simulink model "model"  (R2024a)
settings: Solver=VariableStepAuto  StartTime=0.0  StopTime=7*3600  RelTol=1e-3
libraries: fl_lib x8, nesl_utility x2, batteryecm_lib x1

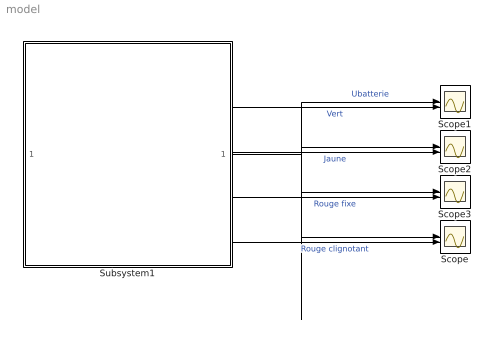
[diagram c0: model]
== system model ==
  Scope{,1..3} (4 alike) : Scope  NumInputPorts=2
  Subsystem1 : Subsystem  mask{U=0, Q=0}
      mask prompts: U "Tension batterie (V)"; Q "Capacité A.h)"
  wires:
  Subsystem1/1(Ubatterie) -> Scope1/1, Scope/1, Scope3/1, Scope2/1  "Ubatterie"
  Subsystem1/2(Vert) -> Scope1/2  "Vert"
  Subsystem1/3(Jaune) -> Scope2/2  "Jaune"
  Subsystem1/4(Rouge fixe) -> Scope3/2  "Rouge fixe"
  Subsystem1/5(Rouge clignotant) -> Scope/2  "Rouge clignotant"

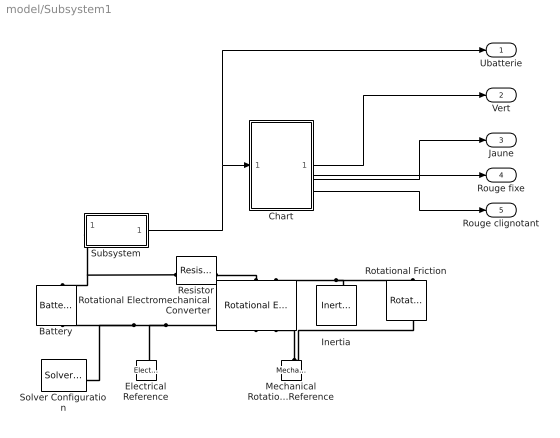
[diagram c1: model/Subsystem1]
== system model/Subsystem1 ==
  Battery : batteryecm_lib/Battery  Vnom=U V  prm_dir=simscape.enum.battery.prm_dir.disabled  R1_dis=2 Ohm  R1_ch=2 Ohm  R1=0.1 Ohm  prm_AH=simscape.enum.battery.prm_AH.finite  AH=Q A*hr  V1=U*0.8 V  AH1=Q*0.2 A*hr  prm_R2=simscape.enum.battery.prm_R2.disabled  R2=2000 Ohm  Tmeas=298.15 K  charge_measurement_port=simscape.enum.battery.enable.no  prm_dyn=simscape.enum.battery.prm_dyn.off  Rp1=0.005 Ohm  tau1=30 s  Rp2=0.005 Ohm  tau2=30 s  Rp3=0.005 Ohm  tau3=30 s  Rp4=0.005 Ohm  tau4=30 s  Rp5=0.005 Ohm  tau5=30 s  prm_fade=simscape.enum.battery.prm_fade.disabled  N_fade=100  AH_fade=45 A*hr  R1_fade=2.02 Ohm  R1_ch_fade=2.02 Ohm  V1_fade=10.35 V  prm_age=simscape.enum.battery.prm_age.disabled  prm_age_OCV=simscape.enum.battery.prm_age_OCV.OCV  OCV_age=0.9  SOC_age=60  Tmeas_age=298.15 K  delta_time_age_vec=[0] d  temperature_age_vec=[273] K  OCV_scaling_age=2.2134e6  OCV_offset_age=1.632e6  temp_exp_age=0.515833569 V  t_exp_age=0.75  Vnom_T2=12 V  R1_T2=2.2 Ohm  R1_T2_dis=2.2 Ohm  R1_T2_ch=2.2 Ohm  V1_T2=11.4 V  R2_T2=2200 Ohm  Rp1_T2=0.005 Ohm  tau1_T2=30 s  Rp2_T2=0.005 Ohm  tau2_T2=30 s  Rp3_T2=0.005 Ohm  tau3_T2=30 s  Rp4_T2=0.005 Ohm  tau4_T2=30 s  Rp5_T2=0.005 Ohm  tau5_T2=30 s  Tmeas2=273.15 K  thermal_port=simscape.enum.thermaleffects.omit  thermal_mass=30000 J/K  i_specify=off  i_priority=None  i=0 A  i_nominal_specify=off  i_nominal_value=1  i_nominal_unit=A  v_specify=off  v_priority=None  v=0 V  v_nominal_specify=off  v_nominal_value=1  v_nominal_unit=V  charge_specify=off  charge_priority=High  charge=50 A*hr  charge_nominal_specify=off  charge_nominal_value=1  charge_nominal_unit=A*hr  num_cycles_specify=off  num_cycles_priority=High  num_cycles=0  num_cycles_nominal_specify=off  num_cycles_nominal_value=1  num_cycles_nominal_unit=1  temperature_specify=off  temperature_priority=High  temperature=298.15 K  temperature_nominal_specify=off  temperature_nominal_value=1  temperature_nominal_unit=K
  Chart : Stateflow chart  TreatAsAtomicUnit=on
  Electrical Reference : fl_lib/Electrical/Electrical Elements/Electrical Reference
  Inertia : fl_lib/Mechanical/Rotational Elements/Inertia  inertia=0.0001 kg*m^2  num_ports=foundation.enum.numPorts2.one  w_specify=off  w_priority=High  w=0 rad/s  w_nominal_specify=off  w_nominal_value=1  w_nominal_unit=rad/s  t_specify=off  t_priority=None  t=0 N*m  t_nominal_specify=off  t_nominal_value=1  t_nominal_unit=N*m
  Mechanical Rotational Reference : fl_lib/Mechanical/Rotational Elements/Mechanical Rotational Reference
  Resistor : fl_lib/Electrical/Electrical Elements/Resistor  R=0.1 Ohm  i_specify=off  i_priority=None  i=0 A  i_nominal_specify=off  i_nominal_value=1  i_nominal_unit=A  v_specify=off  v_priority=None  v=0 V  v_nominal_specify=off  v_nominal_value=1  v_nominal_unit=V
  Rotational Electromechanical Converter : fl_lib/Electrical/Electrical Elements/Rotational Electromechanical Converter  K=1e-1 V*s/rad  i_specify=off  i_priority=None  i=0 A  i_nominal_specify=off  i_nominal_value=1  i_nominal_unit=A  v_specify=off  v_priority=None  v=0 V  v_nominal_specify=off  v_nominal_value=1  v_nominal_unit=V  t_specify=off  t_priority=None  t=0 N*m  t_nominal_specify=off  t_nominal_value=1  t_nominal_unit=N*m  w_specify=off  w_priority=None  w=0 rad/s  w_nominal_specify=off  w_nominal_value=1  w_nominal_unit=rad/s
  Rotational Friction : fl_lib/Mechanical/Rotational Elements/Rotational Friction  brkwy_trq=1e-5 N*m  brkwy_vel=1e-5 rad/s  Col_trq=1e-5 N*m  visc_coef=1.5e-2 N*m*s/rad  w_specify=off  w_priority=None  w=0 rad/s  w_nominal_specify=off  w_nominal_value=1  w_nominal_unit=rad/s  t_specify=off  t_priority=None  t=0 N*m  t_nominal_specify=off  t_nominal_value=1  t_nominal_unit=N*m
  Solver Configuration : nesl_utility/Solver Configuration  PhysicalDomain=network_engine_domain  SubClassName=solver  LeftPortType=input  RightPortType=generic  Tones=[]  Harmonics=[]  SimulateNoise=off  Profile=off  UseLocalSampling=off  EnableSwitchedLinearOptims=on  FrequencyDomain=off  UseCCode=off  RelTol=0.001  AbsTol=0.001  MinStep=1e-09  ToWorkspace=off  RevertToSquareIcSolve=off  NumHomotopyIterations=100  PhasorMode=off  PhasorModeNumHarmonics=1  ConsistencySolver=NEWTON_XTOL_AFTER_FTOL  IndexReductionMethod=DerivativeReplacement  DoDC=off  ResidualTolerance=1e-09  ConsistencyTolSource=GLOBAL  ConsistencyAbsTol=0.001  ConsistencyRelTol=0.001  ConsistencyTolFactor=0.001  UseLocalSolver=off  LocalSolverChoice=NE_BACKWARD_EULER_ADVANCER  ResolveIndetEquations=on  FunctionEvalNumThread=1  LocalSolverSampleTime=0.001  DoFixedCost=off  MaxNonlinIter=3  MaxModeIter=2  ComputeImpulses=off  ImpulseIterations=2  LinearAlgebra=auto  LinearAlgebraNumThread=0  EquationFormulation=NE_TIME_EF  DelaysMemoryBudget=1024  AutomaticFiltering=off  FilteringTimeConstant=0.001  PartitionStorageMethod=AS_NEEDED  PartitionMemoryBudget=1024  PartitionMethod=ROBUST  MultibodyUseLocalSolver=off  MultibodyLocalSolverChoice=ODE1  MultibodyLocalSolverSampleTime=0.001
  Subsystem : Subsystem
  Ubatterie : Outport
  Vert : Outport  Port=2
  Jaune : Outport  Port=3
  Rouge fixe : Outport  Port=4
  Rouge clignotant : Outport  Port=5
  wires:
  Chart/1(led1) -> Vert/1
  Subsystem/1(output) -> Ubatterie/1, Chart/1(tension)
  Chart/4(led4) -> Rouge clignotant/1
  Chart/3(led3) -> Rouge fixe/1
  Chart/2(led2) -> Jaune/1
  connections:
  Rotational Electromechanical Converter/LConn2 -- Inertia/LConn1 -- Rotational Friction/LConn1
  Mechanical Rotational Reference/LConn1 -- Rotational Electromechanical Converter/RConn2 -- Rotational Friction/RConn1
  Rotational Electromechanical Converter/LConn1 -- Resistor/RConn1
  Subsystem/LConn1 -- Resistor/LConn1 -- Battery/LConn1
  Rotational Electromechanical Converter/RConn1 -- Electrical Reference/LConn1 -- Solver Configuration/RConn1 -- Battery/RConn1

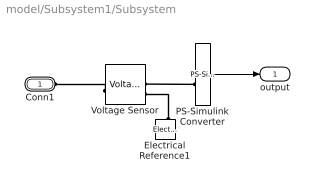
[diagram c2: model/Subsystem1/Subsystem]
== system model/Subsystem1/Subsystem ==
  Electrical Reference1 : fl_lib/Electrical/Electrical Elements/Electrical Reference
  PS-Simulink Converter : nesl_utility/PS-Simulink Converter  PhysicalDomain=network_engine_domain  SubClassName=ps_output  LeftPortType=input  RightPortType=output  PseudoPeriodic=off  Frequencies=[]  VectorFormat=inherit  Unit=inherit  AffineConversion=off
  Voltage Sensor : fl_lib/Electrical/Electrical Sensors/Voltage Sensor
  Conn1 : PMIOPort  Side=Left
  output : Outport
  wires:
  PS-Simulink Converter/1 -> output/1
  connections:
  Voltage Sensor/LConn1 -- Conn1/RConn1
  PS-Simulink Converter/LConn1 -- Voltage Sensor/RConn1
  Electrical Reference1/LConn1 -- Voltage Sensor/RConn2

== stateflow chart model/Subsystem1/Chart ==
  state charge1
    entry: led1=1
    exit : led1=0
  state charge2
    entry: led2=1
    exit: led2=0
  state charge3
    entry: led3=1
    exit: led3=0
  state charge4
    entry: led4=1
    exit: led4=0
  (default) -> charge1
  charge3 -> charge2 : [tension>7]
  charge2 -> charge1 : [tension>(8) ]
  charge4 -> charge3 : [tension>6.7]
  charge2 -> charge3 : [tension<6.95]
  charge1 -> charge2 : [tension<7.95]
  charge3 -> charge4 : [tension<6.65]
  data: led1 output; led2 output; tension input; led3 output; led4 output
